| IBIS file stm32l552_562_lqfp48.ibs
[IBIS ver]   4.2
[File name]  stm32l552_562_lqfp48.ibs
[File Rev]   1.0
[Date]   04-10-2019
[Source]   Data Created at STMicroelectronics
[Notes]   File originated from ELDO simulations.
[Disclaimer] This information is for modeling purpose only and is
   not guaranted.
   The information is subject to change without notice.
[Copyright]  Copyright 2019 STMicroelectronics Inc.
|   Component stm32l552_562_lqfp48
[Component] stm32l552_562_lqfp48
[Manufacturer] STMicroelectronics
[Package]
| variable   typ   min   max
R_pkg  0  NA  NA
L_pkg  0  NA  NA
C_pkg  0  NA  NA
[Pin]   signal_name   model_name R_pin L_pin C_pin
1 VBAT POWER 0.053 3.42534E-09 9.041E-14
2 PC13 io8prog2m25m50m120m_sudq_ft 0.048377332 2.91404E-09 6.443E-14
3 PC14-OSC32_IN io8prog2m25m50m120m_sudq_ft 0.044678997 2.50442E-09 4.365E-14
4 PC15-OSC32_OUT io8prog2m25m50m120m_sudq_ft 0.041905328 2.19704E-09 2.807E-14
5 PH0-OSC_IN io8prog2m25m50m120m_sudq_ft 0.040056325 1.9919E-09 1.769E-14
6 PH1-OSC_OUT io8prog2m25m50m120m_sudq_ft 0.03913 1.89021E-09 1.24625E-14
7 NRST ioreset_ft_v33 0.03913 1.89021E-09 1.24625E-14
8 VSSA_VREF- GND 0.040057312 1.98992E-09 1.775E-14
9 VDDA_VREF+ POWER 0.041906973 2.19374E-09 2.817E-14
10 PA0 io8prog2m25m50m120m_sudq_ft 0.0446813 2.4998E-09 4.379E-14
11 PA1 io8prog2m25m50m120m_sudq_ft 0.048380293 2.9081E-09 6.461E-14
12 PA2 io8prog2m25m50m120m_sudq_ft 0.053 3.42534E-09 9.041E-14
13 PA3 io8prog2m25m50m120m_sudq_ft 0.053 3.42534E-09 9.041E-14
14 PA4 io8prog2m25m50m120m_sudq_ft 0.048377332 2.91404E-09 6.443E-14
15 PA5 io8prog2m25m50m120m_sudq_ft 0.044678997 2.50442E-09 4.365E-14
16 PA6 io8prog2m25m50m120m_sudq_ft 0.041905328 2.19704E-09 2.807E-14
17 PA7 io8prog2m25m50m120m_sudq_i2c_ft 0.040056325 1.9919E-09 1.769E-14
18 PB0 io8prog2m25m50m120m_sudq_ft 0.03913 1.89021E-09 1.24625E-14
19 PB1 io8prog2m25m50m120m_sudq_ft 0.03913 1.89021E-09 1.24625E-14
20 PB2 io8prog2m25m50m120m_sudq_ft 0.040057312 1.98992E-09 1.775E-14
21 PB10 io8prog2m25m50m120m_sudq_i2c_ft 0.041906973 2.19374E-09 2.817E-14
22 PB11 io8prog2m25m50m120m_sudq_i2c_ft 0.0446813 2.4998E-09 4.379E-14
23 VSS GND 0.048380293 2.9081E-09 6.461E-14
24 VDD POWER 0.053 3.42534E-09 9.041E-14
25 PB12 io8prog2m25m50m120m_sudq_ft 0.053 3.42534E-09 9.041E-14
26 PB13 io8prog2m25m50m120m_sudq_i2c_ft 0.048377332 2.91404E-09 6.443E-14
27 PB14 io8prog2m25m50m120m_sudq_i2c_ft 0.044678997 2.50442E-09 4.365E-14
28 PB15 io6usb_bmc_pd_cc_ft 0.041905328 2.19704E-09 2.807E-14
29 PA8 io8prog2m25m50m120m_sudq_i2c_ft 0.040056325 1.9919E-09 1.769E-14
30 PA9 io8prog2m25m50m120m_sudq_ft 0.03913 1.89021E-09 1.24625E-14
31 PA10 io8prog2m25m50m120m_sudq_ft 0.03913 1.89021E-09 1.24625E-14
32 PA11 io8usblsfs_otg2 0.040057312 1.98992E-09 1.775E-14
33 PA12 io8usblsfs_otg2 0.041906973 2.19374E-09 2.817E-14
34 PA13 io8prog2m25m50m120m_sudq_ft 0.0446813 2.4998E-09 4.379E-14
35 VSS GND 0.048380293 2.9081E-09 6.461E-14
36 VDD POWER 0.053 3.42534E-09 9.041E-14
37 PA14 io8prog2m25m50m120m_sudq_i2c_ft 0.053 3.42534E-09 9.041E-14
38 PA15 io6usb_bmc_pd_cc_ft 0.048377332 2.91404E-09 6.443E-14
39 PB3 io8prog2m25m50m120m_sudq_ft 0.044678997 2.50442E-09 4.365E-14
40 PB4 io8prog2m25m50m120m_sudq_i2c_ft 0.041905328 2.19704E-09 2.807E-14
41 PB5 io8prog2m25m50m120m_sudq_ft 0.040056325 1.9919E-09 1.769E-14
42 PB6 io8prog2m25m50m120m_sudq_i2c_ft 0.03913 1.89021E-09 1.24625E-14
43 PB7 io8prog2m25m50m120m_sudq_i2c_ft 0.03913 1.89021E-09 1.24625E-14
44 PH3-BOOT0 io8prog2m25m50m120m_sudq_ft 0.040057312 1.98992E-09 1.775E-14
45 PB8 io8prog2m25m50m120m_sudq_i2c_ft 0.041906973 2.19374E-09 2.817E-14
46 PB9 io8prog2m25m50m120m_sudq_i2c_ft 0.0446813 2.4998E-09 4.379E-14
47 VSS GND 0.048380293 2.9081E-09 6.461E-14
48 VDD POWER 0.053 3.42534E-09 9.041E-14
[Model Selector] io6usb_bmc_pd_cc_ft
usb_bmc_emit_pdccpd  "BMC PD emitter  + PD"
usb_bmc_emit_pdcc3a0  "BMC PD emitter  + 3rd PU"
usb_bmc_emit_pdcc1a5  "BMC PD emitter  + 2nd PU"
usb_bmc_emit_pdccusb  "BMC PD emitter  + 1st PU"
usb_bmc_emit  "BMC PD emitter "
io2_pdcc_ft_3v3_lowspeed  "GPIO-3.3V range - low speed"
io2_pdcc_ft_3v3_mediumspeed  "GPIO-3.3V range - medium speed"
io2_pdcc_ft_3v3_lowspeed_pu  "GPIO-3.3V range - low speed - pull up"
io2_pdcc_ft_3v3_mediumspeed_pu  "GPIO-3.3V range - medium speed - pull up"
io2_pdcc_ft_3v3_lowspeed_pd  "GPIO-3.3V range - low speed - pull down"
io2_pdcc_ft_3v3_mediumspeed_pd  "GPIO-3.3V range - medium speed - pull down"
io2_pdcc_ft_1v8_lowspeed  "GPIO-1.8V range - low speed"
io2_pdcc_ft_1v8_mediumspeed  "GPIO-1.8V range - medium speed"
io2_pdcc_ft_1v8_lowspeed_pu  "GPIO-1.8V range - low speed - pull up"
io2_pdcc_ft_1v8_mediumspeed_pu  "GPIO-1.8V range - medium speed - pull up"
io2_pdcc_ft_1v8_lowspeed_pd  "GPIO-1.8V range - low speed - pull down"
io2_pdcc_ft_1v8_mediumspeed_pd  "GPIO-1.8V range - medium speed - pull down"
io2_pdcc_ft_1v2_lowspeed  "GPIO-1.2V range - low speed"
io2_pdcc_ft_1v2_mediumspeed  "GPIO-1.2V range - medium speed"
io2_pdcc_ft_1v2_lowspeed_pu  "GPIO-1.2V range - low speed - pull up"
io2_pdcc_ft_1v2_mediumspeed_pu  "GPIO-1.2V range - medium speed - pull up"
io2_pdcc_ft_1v2_lowspeed_pd  "GPIO-1.2V range - low speed - pull down"
io2_pdcc_ft_1v2_mediumspeed_pd  "GPIO-1.2V range - medium speed - pull down"
[Model Selector] io8prog2m25m50m120m_sudq_ft
iols8p_sudq_ft_pd_lv  "IO low speed, PD=40kOhm - 1P8V"
iols8p_sudq_ft_pu_lv  "IO low speed, PU=40kOhm - 1P8V"
iols8p_sudq_ft_lv  "IO low speed - 1P8V"
iols8p_sudq_ft_pd  "IO low speed, PD=40kOhm - 3P3V"
iols8p_sudq_ft_pu  "IO low speed, PU=40kOhm - 3P3V"
iols8p_sudq_ft  "IO low speed - 3P3V"
iofs8p_sudq_ft_pd_lv  "IO full speed, PD=40kOhm - 1P8V"
iofs8p_sudq_ft_pu_lv  "IO full speed, PU=40kOhm - 1P8V"
iofs8p_sudq_ft_lv  "IO full speed - 1P8V"
iofs8p_sudq_ft_pd  "IO full speed, PD=40kOhm - 3P3V"
iofs8p_sudq_ft_pu  "IO full speed, PU=40kOhm - 3P3V"
iofs8p_sudq_ft  "IO full speed - 3P3V"
ioms8p_sudq_ft_pd_lv  "IO medium speed, PD=40kOhm - 1P8V"
ioms8p_sudq_ft_pu_lv  "IO medium speed, PU=40kOhm - 1P8V"
ioms8p_sudq_ft_lv  "IO medium speed - 1P8V"
ioms8p_sudq_ft_pd  "IO medium speed, PD=40kOhm - 3P3V"
ioms8p_sudq_ft_pu  "IO medium speed, PU=40kOhm - 3P3V"
ioms8p_sudq_ft  "IO medium speed - 3P3V"
iohs8p_sudq_ft_pd_lv  "IO high speed, PD=40kOhm - 1P8V"
iohs8p_sudq_ft_pu_lv  "IO high speed, PU=40kOhm - 1P8V"
iohs8p_sudq_ft_lv  "IO high speed - 1P8V"
iohs8p_sudq_ft_pd  "IO high speed, PD=40kOhm - 3P3V"
iohs8p_sudq_ft_pu  "IO high speed, PU=40kOhm - 3P3V"
iohs8p_sudq_ft  "IO high speed - 3P3V"
[Model Selector] io8prog2m25m50m120m_sudq_i2c_ft
io8prog_1v8_i2c_pd  "5V Tol GPIO 1.8V range i2c functionality with pull down"
io8prog_1v8_i2c_pu  "5V Tol GPIO 1.8V range i2c functionality with pull up"
io8prog_1v8_i2c  "5V Tol GPIO 1.8V range i2c functionality"
io8prog_3v3_i2c_pd  "5V Tol GPIO 3.3V range i2c functionality with pull down"
io8prog_3v3_i2c_pu  "5V Tol GPIO 3.3V range i2c functionality with pull up"
io8prog_3v3_i2c  "5V Tol GPIO 3.3V range i2c functionality"
iols8p_sudq_ft_pd_lv  "IO low speed, PD=40kOhm - 1P8V"
iols8p_sudq_ft_pu_lv  "IO low speed, PU=40kOhm - 1P8V"
iols8p_sudq_ft_lv  "IO low speed - 1P8V"
iols8p_sudq_ft_pd  "IO low speed, PD=40kOhm - 3P3V"
iols8p_sudq_ft_pu  "IO low speed, PU=40kOhm - 3P3V"
iols8p_sudq_ft  "IO low speed - 3P3V"
iofs8p_sudq_ft_pd_lv  "IO full speed, PD=40kOhm - 1P8V"
iofs8p_sudq_ft_pu_lv  "IO full speed, PU=40kOhm - 1P8V"
iofs8p_sudq_ft_lv  "IO full speed - 1P8V"
iofs8p_sudq_ft_pd  "IO full speed, PD=40kOhm - 3P3V"
iofs8p_sudq_ft_pu  "IO full speed, PU=40kOhm - 3P3V"
iofs8p_sudq_ft  "IO full speed - 3P3V"
ioms8p_sudq_ft_pd_lv  "IO medium speed, PD=40kOhm - 1P8V"
ioms8p_sudq_ft_pu_lv  "IO medium speed, PU=40kOhm - 1P8V"
ioms8p_sudq_ft_lv  "IO medium speed - 1P8V"
ioms8p_sudq_ft_pd  "IO medium speed, PD=40kOhm - 3P3V"
ioms8p_sudq_ft_pu  "IO medium speed, PU=40kOhm - 3P3V"
ioms8p_sudq_ft  "IO medium speed - 3P3V"
iohs8p_sudq_ft_pd_lv  "IO high speed, PD=40kOhm - 1P8V"
iohs8p_sudq_ft_pu_lv  "IO high speed, PU=40kOhm - 1P8V"
iohs8p_sudq_ft_lv  "IO high speed - 1P8V"
iohs8p_sudq_ft_pd  "IO high speed, PD=40kOhm - 3P3V"
iohs8p_sudq_ft_pu  "IO high speed, PU=40kOhm - 3P3V"
iohs8p_sudq_ft  "IO high speed - 3P3V"
[Model Selector] io8usblsfs_otg2
usb_ls_pd  "USB Low Speed mode - Pull Down"
usb_ls_pu2  "USB Low Speed mode - Pull up 2"
usb_ls_pu  "USB Low Speed mode - Pull up"
usb_fs  "USB Low Speed mode"
usb_fs_pd  "USB Full Speed mode - Pull Down"
usb_fs_pu2  "USB Full Speed mode - Pull up 2"
usb_fs_pu  "USB Full Speed mode - Pull up"
[Model Selector] ioreset_ft_v33
ioreset_1v2_pu  "RESET 1.2V range with PU"
ioreset_1v2  "RESET 1.2V range"
ioreset_1v8_pu  "RESET 1.8V range with PU"
ioreset_1v8  "RESET 1.8V range"
ioreset_3v3_pu  "RESET 3.3V range with PU"
ioreset_3v3  "RESET 3.3V range"
| Models and submodels in the file (66): usb_bmc_emit_pdccpd (I/O), usb_bmc_emit_pdcc3a0 (I/O), usb_bmc_emit_pdcc1a5 (I/O), usb_bmc_emit_pdccusb (I/O), usb_bmc_emit (I/O), io2_pdcc_ft_3v3_lowspeed (I/O), io2_pdcc_ft_3v3_mediumspeed (I/O), io2_pdcc_ft_3v3_lowspeed_pu (I/O), io2_pdcc_ft_3v3_mediumspeed_pu (I/O), io2_pdcc_ft_3v3_lowspeed_pd (I/O), io2_pdcc_ft_3v3_mediumspeed_pd (I/O), io2_pdcc_ft_1v8_lowspeed (I/O), io2_pdcc_ft_1v8_mediumspeed (I/O), io2_pdcc_ft_1v8_lowspeed_pu (I/O), io2_pdcc_ft_1v8_mediumspeed_pu (I/O), io2_pdcc_ft_1v8_lowspeed_pd (I/O), io2_pdcc_ft_1v8_mediumspeed_pd (I/O), io2_pdcc_ft_1v2_lowspeed (I/O), io2_pdcc_ft_1v2_mediumspeed (I/O), io2_pdcc_ft_1v2_lowspeed_pu (I/O), io2_pdcc_ft_1v2_mediumspeed_pu (I/O), io2_pdcc_ft_1v2_lowspeed_pd (I/O), io2_pdcc_ft_1v2_mediumspeed_pd (I/O), iols8p_sudq_ft_pd_lv (I/O), iols8p_sudq_ft_pu_lv (I/O), iols8p_sudq_ft_lv (I/O), iols8p_sudq_ft_pd (I/O), iols8p_sudq_ft_pu (I/O), iols8p_sudq_ft (I/O), iofs8p_sudq_ft_pd_lv (I/O), iofs8p_sudq_ft_pu_lv (I/O), iofs8p_sudq_ft_lv (I/O), iofs8p_sudq_ft_pd (I/O), iofs8p_sudq_ft_pu (I/O), iofs8p_sudq_ft (I/O), ioms8p_sudq_ft_pd_lv (I/O), ioms8p_sudq_ft_pu_lv (I/O), ioms8p_sudq_ft_lv (I/O), ioms8p_sudq_ft_pd (I/O), ioms8p_sudq_ft_pu (I/O), ioms8p_sudq_ft (I/O), iohs8p_sudq_ft_pd_lv (I/O), iohs8p_sudq_ft_pu_lv (I/O), iohs8p_sudq_ft_lv (I/O), iohs8p_sudq_ft_pd (I/O), iohs8p_sudq_ft_pu (I/O), iohs8p_sudq_ft (I/O), io8prog_1v8_i2c_pd (I/O_open_drain), io8prog_1v8_i2c_pu (I/O_open_drain), io8prog_1v8_i2c (I/O_open_drain), io8prog_3v3_i2c_pd (I/O_open_drain), io8prog_3v3_i2c_pu (I/O_open_drain), io8prog_3v3_i2c (I/O_open_drain), usb_ls_pd (I/O), usb_ls_pu2 (I/O), usb_ls_pu (I/O), usb_fs (I/O), usb_fs_pd (I/O), usb_fs_pu2 (I/O), usb_fs_pu (I/O), ioreset_1v2_pu (I/O_open_drain), ioreset_1v2 (I/O_open_drain), ioreset_1v8_pu (I/O_open_drain), ioreset_1v8 (I/O_open_drain), ioreset_3v3_pu (I/O_open_drain), ioreset_3v3 (I/O_open_drain)
